TYPE VG_INPUT :
STRUCT
		Reading_Valid:BOOL;
		Overrange_Exceeded:BOOL;
		Underrange_Exceeded:BOOL;
		Sensor_Value:REAL;
		Reading_Valid_1:BOOL;
		Overrange_Exceeded_1:BOOL;
		Underrange_Exceeded_1:BOOL;
		Sensor_Value_1:REAL;
		Active_Exception_Status_2:USINT;
		Trip_Point_Output_All_Insta_2:UDINT;
		Active_Device_Warning_Details:UDINT;
		Active_Device_Error_Details:UDINT;
END_STRUCT
END_TYPE
